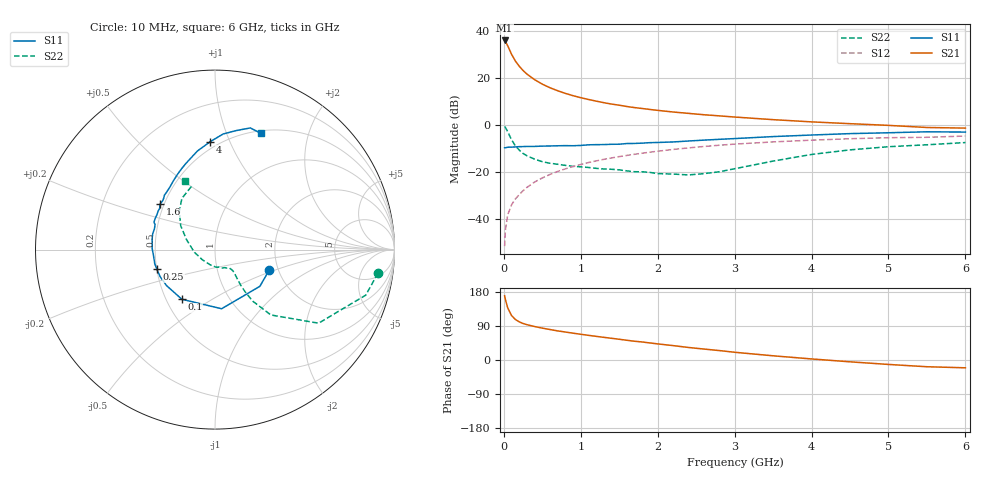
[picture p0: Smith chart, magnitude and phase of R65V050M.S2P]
! SIEMENS Small Signal Semiconductors
! BFR193
! Si NPN RF Bipolar Junction Transistor in SOT23
! VCE = 5 V  IC = 50 mA
! Common Emitter S-Parameters:  May  1996
# GHz  S  MA  R  50
!  f  S11  S21  S12  S22
! GHz  MAG  ANG  MAG  ANG  MAG  ANG  MAG  ANG
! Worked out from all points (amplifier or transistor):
!   36 points, 10 MHz to 6 GHz, reference 50 ohm
!   highest |S21| = 35.8 dB at 10 MHz (marker M1)
!   |S21| within 3 dB of that: start of sweep to 60.3 MHz
!   unconditionally stable (mu >= 1): 420 MHz to 2.065 GHz
!   at 250 MHz: K = 0.95, MSG = 25.6 dB, |S12| = -28.1 dB
!   at 1.4 GHz: K = 1.02, MAG = 10.6 dB, |S12| = -14.2 dB
!   at 6 GHz: K = 0.95, MSG = 1.7 dB, |S12| = -4.8 dB
!   S11 on the Smith chart (normalised r, x): 10 MHz: 1.79, -0.46; 100 MHz: 0.60, -0.37; 250 MHz: 0.50, -0.12; 1.6 GHz: 0.48, +0.28; 4 GHz: 0.45, +0.85; 6 GHz: 0.53, +1.33
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0.01  0.3228 -20.7  61.97 169.5  0.0026 80.9  0.9173 -8.2
0.02  0.3231 -39.3  59.3 159.9  0.0057 75.6  0.8775 -16.8
0.05  0.3316 -83.6  47.78 137.7  0.012 70.6  0.7079 -35.4
0.1  0.3327 -123.7  31.57 117.4  0.0197 69.2  0.4788 -49.5
0.15  0.3362 -143.3  22.63 106.9  0.0263 69.4  0.3556 -53.8
0.2  0.3408 -153.7  17.56 100.7  0.0324 71.2  0.2882 -54.5
0.25  0.342 -161.3  14.2 96.3  0.0394 72.2  0.2441 -54.1
0.3  0.3447 -166.9  11.94 93.2  0.0463 73.5  0.2182 -53.3
0.4  0.3447 -175.2  9.078 88.3  0.0602 73.7  0.1846 -51.5
0.5  0.35 179.1  7.284 84.1  0.0736 74.1  0.1631 -50.1
0.6  0.3524 174.1  6.106 80.4  0.0874 73.3  0.1511 -50.0
0.7  0.3558 169.3  5.273 76.8  0.1012 72.5  0.1439 -50.4
0.9  0.3565 161.5  4.137 70.8  0.1292 70.2  0.13 -52.1
1.1  0.3728 155.8  3.439 65.1  0.1564 67.9  0.1229 -56.8
1.3  0.3773 149.0  2.938 59.8  0.183 65.0  0.1141 -61.9
1.6  0.3971 140.6  2.435 52.0  0.222 60.7  0.104 -73.9
2.2  0.4293 125.9  1.861 38.0  0.2972 51.8  0.089 -108.2
3.5  0.5581 100.1  1.279 11.1  0.4298 31.4  0.1679 160.8
4  0.6026 92.4  1.148 2.8  0.4684 24.4  0.2327 145.2
4.5  0.6456 86.0  1.05 -4.8  0.5026 17.3  0.2912 133.0
5.5  0.706 73.8  0.871 -17.8  0.539 3.7  0.3736 111.0
6  0.6961 68.5  0.846 -20.6  0.5735 -0.2  0.4165 113.3
